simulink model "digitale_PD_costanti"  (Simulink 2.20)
settings: Solver=VariableStepDiscrete  StartTime=0.0  StopTime=10.0  RelTol=1e-3  AbsTol=1e-6
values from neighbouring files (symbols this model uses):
  N = 10    [pidin.m]
  Td = 0.1    [pidin.m]
undefined symbols (not defined in the file or in its folder): Kp, T

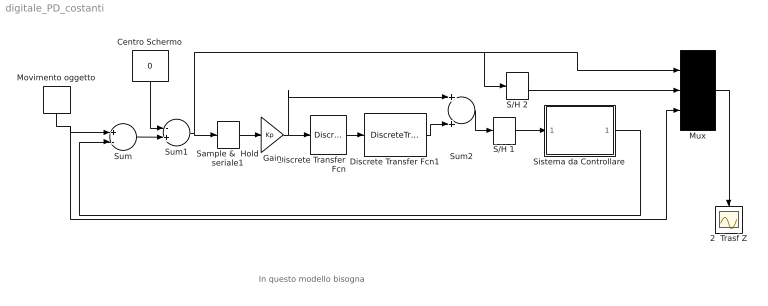
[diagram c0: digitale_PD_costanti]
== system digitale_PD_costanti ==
  note: In questo modello bisogna
  2  Trasf Z : Scope
  Centro Schermo : Constant  Orientation=down  Value=0
  Discrete Transfer Fcn : DiscreteTransferFcn  Numerator=[Td]  Denominator=[ T+Td/N]  SampleTime=0.005
  Discrete Transfer Fcn1 : DiscreteTransferFcn  Numerator=[1 -1]  Denominator=[1 -Td/(N*T+Td)]  SampleTime=.005
  Gain : Gain  Gain=Kp
  Movimento oggetto : DiscretePulseGenerator  Orientation=down  Amplitude=47.5  Period=100  PulseWidth=100  PhaseDelay=10  SampleTime=.1
  Mux : Mux  Inputs=3
  S/H 1 : ZeroOrderHold  SampleTime=.260
  S/H 2 : ZeroOrderHold  SampleTime=.260
  Sample &  Hold seriale1 : ZeroOrderHold  SampleTime=T
  Sistema da Controllare : Subsystem
  Sum : Sum  Inputs=+-
  Sum1 : Sum  Inputs=-+
  Sum2 : Sum  Inputs=++
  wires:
  Sum/1 -> Sum1/2
  Centro Schermo/1 -> Sum1/1
  Mux/1 -> 2  Trasf Z/1
  Sum1/1 -> Sample &  Hold seriale1/1, Mux/1, S/H 2/1
  Discrete Transfer Fcn/1 -> Discrete Transfer Fcn1/1
  Sistema da Controllare/1(Out1) -> Sum/2
  Discrete Transfer Fcn1/1 -> Sum2/2
  Sum2/1 -> S/H 1/1
  Movimento oggetto/1 -> Sum/1, Mux/3
  Gain/1 -> Discrete Transfer Fcn/1, Sum2/1
  Sample &  Hold seriale1/1 -> Gain/1
  S/H 1/1 -> Sistema da Controllare/1(In1)
  S/H 2/1 -> Mux/2

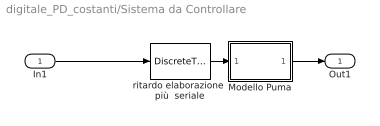
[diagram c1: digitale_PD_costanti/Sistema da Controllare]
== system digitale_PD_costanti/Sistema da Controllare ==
  In1 : Inport  Port=1  PortWidth=-1  SampleTime=-1
  Modello Puma : Subsystem  Description=Modello Puma
  ritardo elaborazione  più  seriale : DiscreteTransferFcn  Numerator=1  Denominator=[1 0 0 0 0 ]  SampleTime=.032
  Out1 : Outport  Port=1
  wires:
  ritardo elaborazione  più  seriale/1 -> Modello Puma/1(In1)
  Modello Puma/1(Out1) -> Out1/1
  In1/1 -> ritardo elaborazione  più  seriale/1

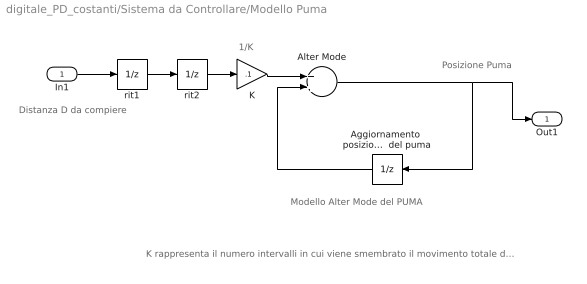
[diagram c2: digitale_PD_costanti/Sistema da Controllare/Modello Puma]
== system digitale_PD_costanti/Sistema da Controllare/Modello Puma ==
  note: Posizione Puma
  note: Modello Alter Mode del PUMA
  note: 1/K
  note: K rappresenta il numero intervalli in cui viene smembrato il movimento totale da compiere, dopo K time-slice (del PUMA) si ottiene che si e' compiuto proprio la distanza D trasmessa.
  note: Distanza D da compiere
  In1 : Inport  Port=1  PortWidth=-1  SampleTime=-1
  Aggiornamento  posizione   Il sample-time di questo blocco rappresenta la TIME-SLICE  del puma : UnitDelay  Orientation=left  X0=0  SampleTime=.032
  Alter Mode : Sum  Inputs=++
  K : Gain  Gain=.1
  rit1 : UnitDelay  X0=0  SampleTime=.032
  rit2 : UnitDelay  X0=0  SampleTime=.032
  Out1 : Outport  Port=1
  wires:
  K/1 -> Alter Mode/1
  Aggiornamento  posizione   Il sample-time di questo blocco rappresenta la TIME-SLICE  del puma/1 -> Alter Mode/2
  Alter Mode/1 -> Out1/1, Aggiornamento  posizione   Il sample-time di questo blocco rappresenta la TIME-SLICE  del puma/1
  In1/1 -> rit1/1
  rit1/1 -> rit2/1
  rit2/1 -> K/1
